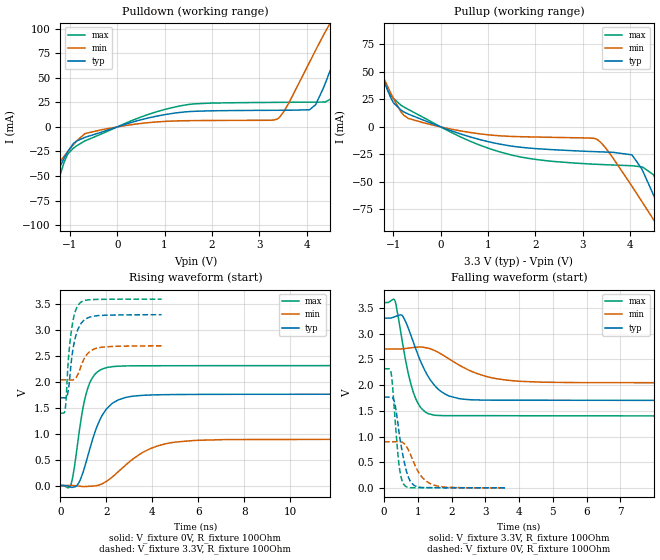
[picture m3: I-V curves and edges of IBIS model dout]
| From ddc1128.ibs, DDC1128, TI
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|   dout Model
[Model]   dout
Model_type   Output
Polarity   Non-Inverting
Vmeas = 1.65
Vref = 0
Cref = 5pF
Rref = 250
|   typ   min   max
|   (nom PVT)   (fast PVT)   (slow PVT)
C_comp   1.593e-12   1.508e-12   1.711e-12
| Where nom  PVT is Nominal Process, 3.3V, 27C
|   Fast PVT is Strong Process,  3.6V, -40C
|   Slow PVT is Weak Process,   2.7V, 125C
[Voltage Range]   3.3   2.7   3.6
|Junction Temperature
[Temperature Range]   27   125   -40
[Pullup Reference]   3.3   2.7   3.6
[Pulldown Reference]   0   0   0
[Power Clamp Reference]   3.3   2.7   3.6
[GND Clamp Reference]   0   0   0
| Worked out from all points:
|   slope of the pulldown table from 0 to 0.495 V, typ, clamps not added: 68.8 ohm
|   slope of the pullup table from 0 to 0.495 V, typ, clamps not added: 66.6 ohm
|   falling waveform, V_fixture 3.3V, R_fixture 100Ohm: 20-80 % time 676ps typ, 1.21ns min, 418ps max; typ from 3.3 V to 1.7 V
|   rising waveform, V_fixture 0V, R_fixture 100Ohm: 20-80 % time 849ps typ, 1.63ns min, 532ps max; typ from 0 V to 1.76 V
|   rising waveform, V_fixture 3.3V, R_fixture 100Ohm: 20-80 % time 340ps typ, 443ps min, 269ps max; typ from 1.69 V to 3.3 V
|   falling waveform, V_fixture 0V, R_fixture 100Ohm: 20-80 % time 274ps typ, 432ps min, 173ps max; typ from 1.77 V to 0.007 V
[Pulldown]
|   Voltage   I(typ)   I(min)   I(max)
-3.3V     -255.8mA   -174.7mA   -389.7mA
-1.67V    -86.07mA   -65.35mA   -120.5mA
-1.059V   -26.34mA   -25.94mA   -29.03mA
-683.7mV  -10.66mA   -6.866mA   -14.26mA
1.252V    14.37mA    6.13mA     20.68mA
3.385V    16.99mA    8.185mA    25.04mA
4.066V    17.49mA    66.1mA     25.25mA
4.192V    22.73mA    78.26mA    25.28mA
4.544V    62.97mA    109.5mA    29.24mA
4.796V    94.04mA    129mA      64.23mA
5.013V    118.7mA    143.7mA    98.61mA
6.6V      221.9mA    211.1mA    239.3mA
[Pullup]
|   Voltage   I(typ)   I(min)   I(max)
-3.3V     203.6mA    184.1mA    223.9mA
-1.729V   103.6mA    93.24mA    118.3mA
-1.09V    29.77mA    33.67mA    30.83mA
-686.4mV  11.71mA    7.75mA     15.93mA
1.251V    -15.65mA   -8.086mA   -22.75mA
3.312V    -22.58mA   -11.65mA   -34.02mA
4.039V    -25.37mA   -53.94mA   -35.28mA
4.494V    -61.84mA   -84.22mA   -43.45mA
4.602V    -72.72mA   -91.47mA   -53.09mA
4.778V    -90.79mA   -103.4mA   -78.44mA
4.864V    -99.67mA   -109.2mA   -91.85mA
6.6V      -281.8mA   -226.6mA   -378.1mA
[Ramp]
R_load = 100
|   typ   min   max
dV/dt_r   1.05814/8.43257e-10   0.536508/1.6286e-09   1.38922/5.30323e-10
dV/dt_f   0.960699/6.7581e-10   0.394003/1.20695e-09   1.32142/4.17693e-10
[Falling Waveform]
V_fixture = 3.3V
V_fixture_min = 2.7V
V_fixture_max = 3.6V
R_fixture = 100Ohm
|   Time   V(typ)   V(min)   V(max)
0s        3.3V       2.7V       3.6V
325ps     3.327V     2.7V       3.634V
550ps     3.342V     2.703V     2.81V
730ps     3.084V     2.717V     2.193V
940ps     2.702V     2.733V     1.736V
1.205ns   2.289V     2.729V     1.488V
1.465ns   2.018V     2.68V      1.419V
2.235ns   1.735V     2.383V     1.406V
3.995ns   1.706V     2.074V     1.405V
14.99ns   1.699V     2.043V     1.398V
[Rising Waveform]
V_fixture = 0V
V_fixture_min = 0V
V_fixture_max = 0V
R_fixture = 100Ohm
|   Time   V(typ)   V(min)   V(max)
0s        2.489nV    3.644nV    2.211nV
450ps     -31.11mV   448.6uV    12.31mV
755ps     21.75mV    -7.753mV   836.5mV
1.115ns   452.5mV    -18.11mV   1.768V
1.435ns   946.7mV    -9.331mV   2.109V
1.825ns   1.362V     36.35mV    2.25V
2.81ns    1.697V     385.7mV    2.308V
3.91ns    1.748V     713.6mV    2.312V
4.99ns    1.756V     838.5mV    2.313V
14.99ns   1.764V     894.2mV    2.315V
[Rising Waveform]
V_fixture = 3.3V
V_fixture_min = 2.7V
V_fixture_max = 3.6V
R_fixture = 100Ohm
|   Time   V(typ)   V(min)   V(max)
0s        1.694V     2.04V      1.396V
210ps     1.692V     2.041V     1.484V
255ps     1.703V     2.041V     1.73V
320ps     1.786V     2.04V      2.272V
435ps     2.23V      2.038V     2.845V
570ps     2.699V     2.044V     3.234V
770ps     3.025V     2.156V     3.483V
1.095ns   3.213V     2.496V     3.576V
1.485ns   3.271V     2.639V     3.591V
4.4ns     3.297V     2.696V     3.598V
[Falling Waveform]
V_fixture = 0V
V_fixture_min = 0V
V_fixture_max = 0V
R_fixture = 100Ohm
|   Time   V(typ)   V(min)   V(max)
0s        1.766V     899.2mV    2.316V
210ps     1.768V     899.1mV    2.235V
330ps     1.61V      900.8mV    1.312V
445ps     1.089V     903.4mV    450.6mV
510ps     809.2mV    898.8mV    200.8mV
605ps     491.8mV    858.8mV    58.1mV
730ps     199mV      730.8mV    14.46mV
885ps     55.29mV    493.5mV    8.129mV
1.415ns   8.439mV    74.57mV    9.437mV
3.585ns   6.645mV    5.608mV    6.155mV
